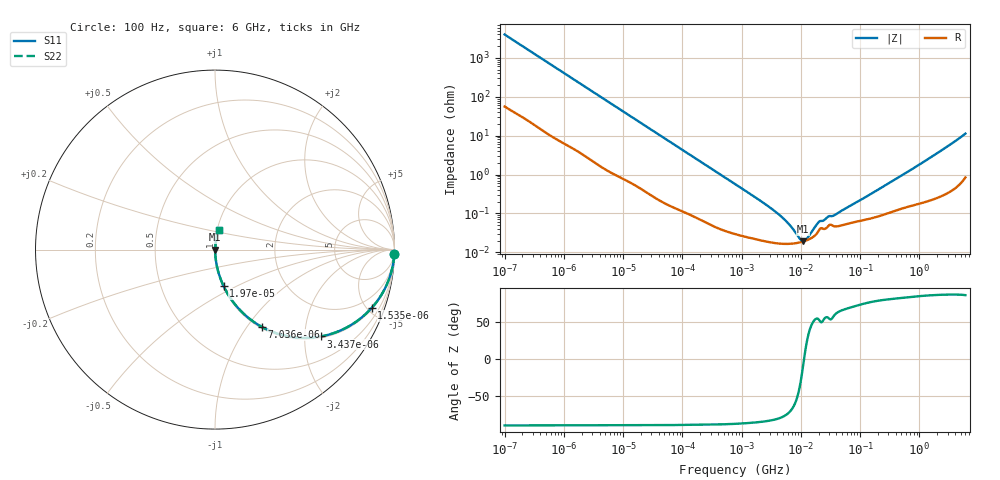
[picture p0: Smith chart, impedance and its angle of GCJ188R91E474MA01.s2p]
!Murata Part Number: GCJ188R91E474MA01
!These Parameters are Measured in Series Mode Connection
!Data Generated on Mar 13, 2026
!  o--ll--o
!Port1  Port2
!  o------o
!Operation Temp=25[degC], DC Bias Voltage=0[V]
!Freq. Start=100[Hz] Stop=6[GHz] 401[Steps]
# Hz S RI R 50
!Freq.(Hz) S11(Real) S11(Imag) S21(Real) S21(Imag) S12(Real) S12(Imag) S22(Real) S22(Imag)
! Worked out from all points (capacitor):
!   401 points, 100 Hz to 6 GHz, reference 50 ohm
!   read as one part in series: C = 397 nF near 109 Hz
!   lowest |Z| = 19.2 mohm at 10.87 MHz (marker M1)
!   series resonance near 11.34 MHz, so ESL is about 500 pH
!   S11 on the Smith chart (normalised r, x): 100 Hz: 2, -80; 1.535 kHz: 1.09, -5.34; 3.437 kHz: 1.04, -2.41; 7.036 kHz: 1.02, -1.18; 19.7 kHz: 1.01, -0.43; 6 GHz: 1.02, +0.22
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100  0.999 -0.025  0.000977 0.025  0.000977 0.025  0.999 -0.025
479  0.9846 -0.1162  0.0154 0.1162  0.0154 0.1162  0.9846 -0.1162
1535  0.873 -0.3249  0.127 0.3249  0.127 0.3249  0.873 -0.3249
2008  0.8034 -0.3892  0.1966 0.3892  0.1966 0.3892  0.8034 -0.3892
3437  0.59 -0.4838  0.41 0.4838  0.41 0.4838  0.59 -0.4838
7036  0.2627 -0.4316  0.7373 0.4316  0.7373 0.4316  0.2627 -0.4316
11514  0.1213 -0.3171  0.8787 0.3171  0.8787 0.3171  0.1213 -0.3171
19704  0.0475 -0.2028  0.9525 0.2028  0.9525 0.2028  0.0475 -0.2028
40335  0.0131 -0.1038  0.9869 0.1038  0.9869 0.1038  0.0131 -0.1038
129199  0.00206 -0.0333  0.9979 0.0333  0.9979 0.0333  0.00206 -0.0333
774597  0.000328 -0.0057  0.9997 0.0057  0.9997 0.0057  0.000328 -0.0057
4246196  0.000169 -0.000932  0.9998 0.000932  0.9998 0.000932  0.000169 -0.000932
6075234  0.000165 -0.000541  0.9998 0.000541  0.9998 0.000541  0.000165 -0.000541
9506416  0.000179 -0.000144  0.9998 0.000144  0.9998 0.000144  0.000179 -0.000144
1.087309e7  0.000189 -3.43e-05  0.9998 3.43e-05  0.9998 3.43e-05  0.000189 -3.43e-05
1.243624e7  0.000203 7.47e-05  0.9998 -7.47e-05  0.9998 -7.47e-05  0.000203 7.47e-05
1.555665e7  0.00024 0.000262  0.9998 -0.000262  0.9998 -0.000262  0.00024 0.000262
2.035112e7  0.000374 0.000487  0.9996 -0.000487  0.9996 -0.000487  0.000374 0.000487
3.80911e7  0.000464 0.000802  0.9995 -0.000802  0.9995 -0.000802  0.000464 0.000802
3.124326e8  0.00107 0.00601  0.9989 -0.00601  0.9989 -0.00601  0.00107 0.00601
1.95892e9  0.00365 0.0343  0.9964 -0.0343  0.9964 -0.0343  0.00365 0.0343
6e9  0.0205 0.1093  0.9795 -0.1093  0.9795 -0.1093  0.0205 0.1093
